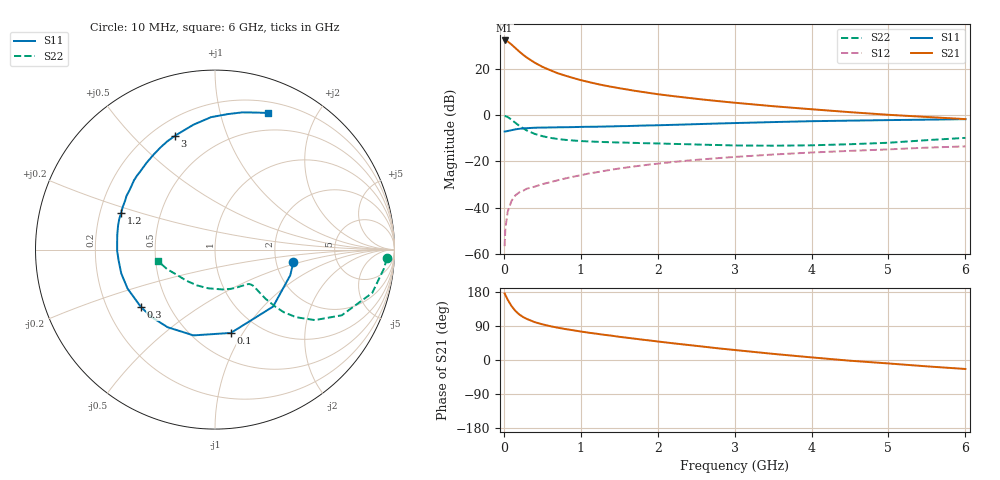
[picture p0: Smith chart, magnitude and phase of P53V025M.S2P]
! SIEMENS Small Signal Semiconductors
! BFP183
! Si NPN RF Bipolar Junction Transistor in SOT143
! VCE = 3 V  IC = 25 mA
! Common Emitter S-Parameters:  March  1996
# GHz  S  MA  R  50
!  f  S11  S21  S12  S22
! GHz  MAG  ANG  MAG  ANG  MAG  ANG  MAG  ANG
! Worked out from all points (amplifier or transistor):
!   36 points, 10 MHz to 6 GHz, reference 50 ohm
!   highest |S21| = 32.1 dB at 10 MHz (marker M1)
!   |S21| within 3 dB of that: start of sweep to 141.2 MHz
!   unconditionally stable (mu >= 1): 691.8 MHz to 5.612 GHz
!   at 250 MHz: K = 0.56, MSG = 29.3 dB, |S12| = -32.6 dB
!   at 1.4 GHz: K = 1.16, MAG = 15.5 dB, |S12| = -23.5 dB
!   at 6 GHz: K = 0.96, MSG = 5.9 dB, |S12| = -13.5 dB
!   S11 on the Smith chart (normalised r, x): 10 MHz: 2.49, -0.44; 100 MHz: 0.74, -0.89; 300 MHz: 0.35, -0.30; 1.2 GHz: 0.29, +0.17; 3 GHz: 0.29, +0.67; 6 GHz: 0.31, +1.42
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0.01  0.4421 -9.3  40.48 175.7  0.0015 81.3  0.958 -2.9
0.02  0.443 -18.9  40.3 171.6  0.0036 84.9  0.9479 -6.3
0.05  0.4534 -44.4  38.53 159.2  0.0083 77.0  0.9087 -15.4
0.1  0.4726 -79.2  33.06 142.3  0.0142 63.3  0.7954 -27.4
0.15  0.4928 -104.1  27.8 129.6  0.0187 56.2  0.6813 -35.2
0.2  0.5066 -121.4  23.43 120.3  0.0216 53.3  0.5888 -39.8
0.25  0.516 -133.2  19.91 113.5  0.0234 51.1  0.5189 -42.3
0.3  0.5221 -142.4  17.29 108.3  0.026 50.2  0.4649 -43.4
0.4  0.5335 -156.0  13.49 100.0  0.0287 51.1  0.3941 -44.2
0.5  0.5389 -165.8  10.97 94.2  0.0325 50.7  0.3516 -44.0
0.6  0.5403 -173.5  9.309 89.4  0.0357 52.7  0.3242 -43.7
0.7  0.5453 -179.3  7.971 85.3  0.0394 53.9  0.3054 -43.5
0.8  0.5469 175.5  7.06 81.6  0.0432 54.8  0.2928 -43.5
1.1  0.5601 162.4  5.169 72.1  0.055 55.7  0.2705 -45.2
1.2  0.5614 158.7  4.73 69.5  0.0584 55.6  0.2664 -46.2
1.7  0.5865 142.1  3.338 56.3  0.0785 53.7  0.2516 -53.6
2.2  0.6158 128.3  2.563 44.1  0.0975 50.2  0.2394 -63.5
3  0.6726 109.3  1.845 26.4  0.1254 43.0  0.2214 -84.6
3.5  0.7065 99.7  1.553 16.2  0.1413 38.6  0.219 -99.9
4.5  0.7587 84.5  1.155 -1.9  0.1694 29.4  0.2356 -132.7
5.5  0.7964 73.5  0.91 -16.8  0.1989 21.3  0.2882 -157.8
6  0.817 68.7  0.819 -23.7  0.2118 16.7  0.3229 -168.4
